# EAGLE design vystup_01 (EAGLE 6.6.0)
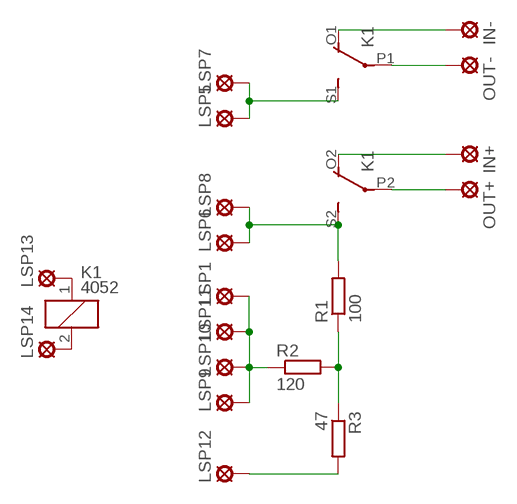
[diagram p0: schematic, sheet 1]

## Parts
IN+  SE14  [SE14]
IN-  SE14  [SE14]
K1  4052  [F4052]
LSP1  SE14  [SE14]
LSP5  SE14  [SE14]
LSP6  SE14  [SE14]
LSP7  SE14  [SE14]
LSP8  SE14  [SE14]
LSP9  SE14  [SE14]
LSP10  SE14  [SE14]
LSP11  SE14  [SE14]
LSP12  SE14  [SE14]
LSP13  SE14  [SE14]
LSP14  SE14  [SE14]
OUT+  SE14  [SE14]
OUT-  SE14  [SE14]
R1  100  R-EU_0207/10  [0207/10]
R2  120  R-EU_0207/10  [0207/10]
R3  47  R-EU_0207/10  [0207/10]

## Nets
GND: LSP1.MP LSP9.MP LSP10.MP LSP11.MP R2.1
N$1: K1.S1(2:S) LSP5.MP LSP7.MP
N$2: K1.S2(3:S) LSP6.MP LSP8.MP R1.2
N$4: K1.P1(2:P) OUT-.MP
N$5: K1.P2(3:P) OUT+.MP
N$6: IN-.MP K1.O1(2:O)
N$7: IN+.MP K1.O2(3:O)
N$8: R1.1 R2.2 R3.1
N$9: LSP12.MP R3.2
N$10: K1.1 LSP13.MP
N$11: K1.2 LSP14.MP

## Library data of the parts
IN+ IN- LSP1 LSP5-LSP14 OUT+ OUT- = solpad:SE14: SOLDER PAD
K1 = relay:4052: RELAY 2 x switch, Finder; OC_FARNELL: unknown; OC_NEWARK: unknown
R1-R3 = rcl:R-EU_: RESISTOR, European symbol

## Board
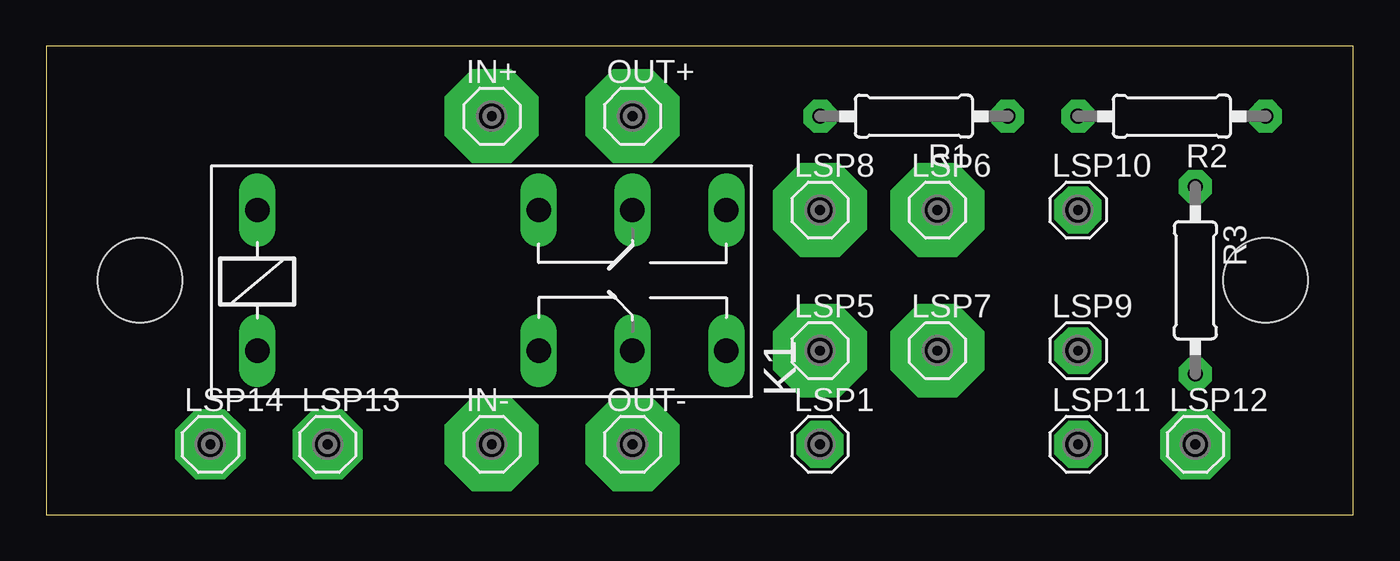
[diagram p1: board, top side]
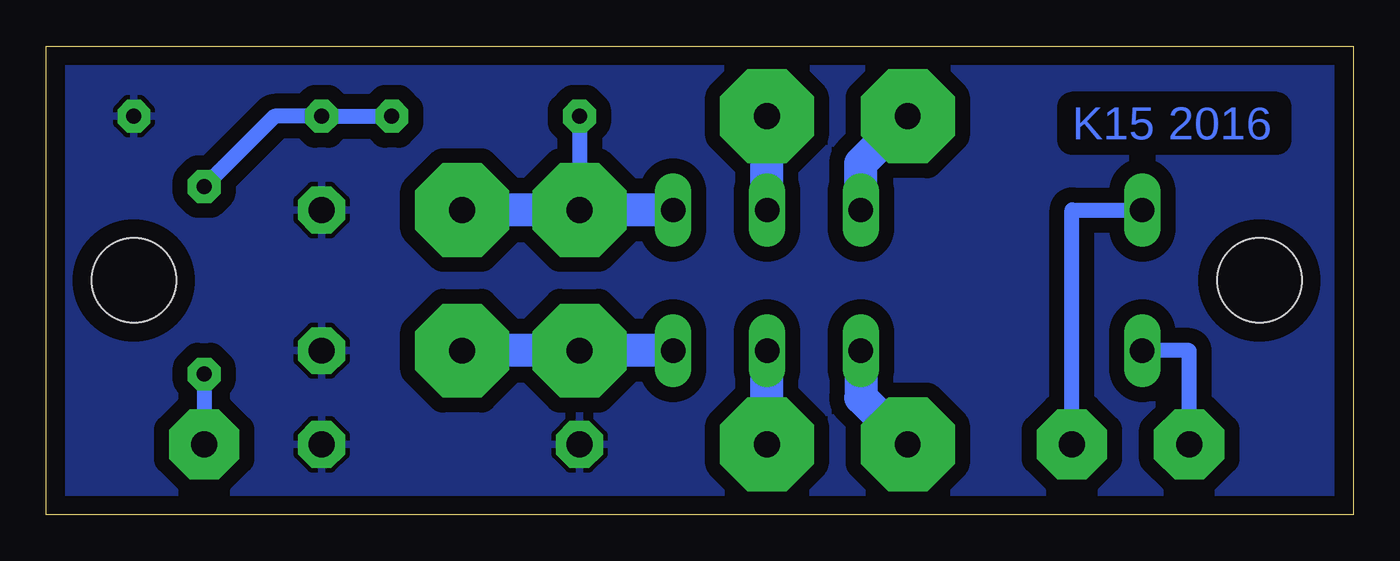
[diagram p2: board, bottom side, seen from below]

Size 70.79 x 25.39 mm. Coordinates in mm from the lower left corner, seen from the top.
Outline: 0,0 70.79,0 70.79,25.39 0,25.39 0,0
Copper layers (1*16): Top 0.035mm / dielectric 1.5mm / Bottom 0.035mm
Design rules "default": minimum track width 10mil, minimum drill 24mil, track to track 8mil, track to pad 8mil, pad to pad 8mil, via to via 8mil, smd to smd 8mil, copper to edge 40mil, drill to drill 8mil, minimum pad ring 10mil, minimum via ring 8mil, stop-mask expansion 4mil, vias tented up to drill 0mil, thermal gap 10mil
Holes 4.57 mm at 5.08,12.7 66.04,12.7

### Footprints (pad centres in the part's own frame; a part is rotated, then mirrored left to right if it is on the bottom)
SE14 = drill 1.397 pad 2.54 octagon: MP 0,0
F4052 = drill 1.321 long: 1 -3.81,3.81; 2 -3.81,-3.81; O1 11.43,-3.81; O2 11.43,3.81; P1 16.51,-3.81; P2 16.51,3.81; S1 21.59,-3.81; S2 21.59,3.81
0207/10 = drill 0.813 pad 1.778 octagon: 1 -5.08,0; 2 5.08,0

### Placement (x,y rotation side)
IN+  24.13,21.59 0 top
IN-  24.13,3.81 0 top
K1  15.24,12.7 0 top
LSP1  41.91,3.81 0 top
LSP5  41.91,8.89 0 top
LSP6  48.26,16.51 0 top
LSP7  48.26,8.89 0 top
LSP8  41.91,16.51 0 top
LSP9  55.88,8.89 0 top
LSP10  55.88,16.51 0 top
LSP11  55.88,3.81 0 top
LSP12  62.23,3.81 0 top
LSP13  15.24,3.81 0 top
LSP14  8.89,3.81 0 top
OUT+  31.75,21.59 0 top
OUT-  31.75,3.81 0 top
R1  46.99,21.59 180 top
R2  60.96,21.59 180 top
R3  62.23,12.7 270 top

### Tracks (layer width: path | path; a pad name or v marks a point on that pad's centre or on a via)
GND
  pour Bottom (isolate 0.813): 0,25.4 71.12,25.4 71.12,0 0,0
N$1  (via drill 0.6 pad 5.08)
  Bottom 1.778: K1.S1 LSP5.MP LSP7.MP
  other vias: 48.26,8.89 41.91,8.89
N$2  (via drill 0.6 pad 5.08)
  Bottom 0.813: R1.2 LSP8.MP
  Bottom 1.778: K1.S2 LSP8.MP LSP6.MP
  other vias: 48.26,16.51 41.91,16.51
N$3  (via drill 0.6 pad 5.08)
  other vias: 24.13,21.59
N$4
  Bottom 1.778: OUT-.MP K1.P1
N$5
  Bottom 1.778: K1.P2 OUT+.MP
N$6
  Bottom 1.778: K1.O1 26.67,6.35 IN-.MP
N$7
  Bottom 1.778: K1.O2 26.67,19.05 IN+.MP
N$8
  Bottom 0.813: R1.1 R2.2 58.42,21.59 R3.1
N$9
  Bottom 0.813: R3.2 LSP12.MP
N$10
  Bottom 0.813: LSP13.MP 15.24,16.51 K1.1
N$11
  Bottom 0.813: LSP14.MP 8.89,8.89 K1.2
N$12  (via drill 0.6 pad 5.08)
  other vias: 31.75,21.59
N$13  (via drill 0.6 pad 5.08)
  other vias: 24.13,3.81
N$14  (via drill 0.6 pad 5.08)
  other vias: 31.75,3.81
N$15  (via drill 0.6 pad 3.81)
  other vias: 15.24,3.81
N$16  (via drill 0.6 pad 3.81)
  other vias: 8.89,3.81
N$17  (via drill 0.6 pad 3.81)
  other vias: 62.23,3.81

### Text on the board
Bottom: K15 2016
